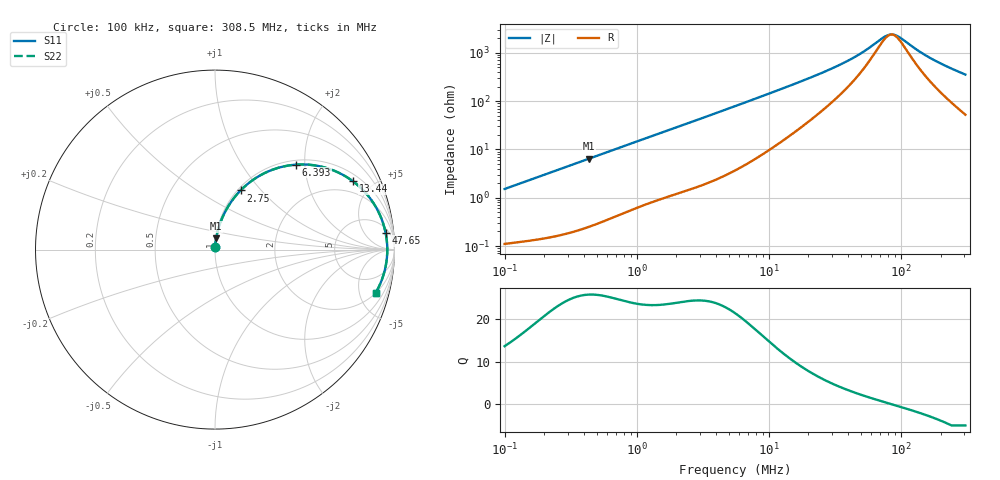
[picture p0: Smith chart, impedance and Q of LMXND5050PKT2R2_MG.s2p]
! LMXND5050PKT2R2_MG  S-PARAMETER MODEL  ( General Type )
! Model Generated by TAIYO YUDEN Corporation (https://www.yuden.co.jp/en/)
! Version 1.0
! TAIYO YUDEN Control No. 191023NI43SB-FBB
! Copyright(c) 2019 TAIYO YUDEN CO.,LTD. All Rights Reserved.
! Product Description (link to TY-COMPAS)
! https://ds.yuden.co.jp/TYCOMPAS/or/detail?pn=LMXND5050PKT2R2NMG&u=M
! Products Name : Inductors
! Characteristics :
!  Inductance : 2.2 uH , SRF(min) : 56 MHz , DC Resistance(max) : 0.078 Ohm
!  Rated Current : Saturation :2800 mA , Temp Rise : 2000 mA (40 degC)
!  Case Size : 4.9 x 4.9 / 0.193 x 0.193 [mm/inch] , Thickness : 1.4 / 0.055 [mm/inch]
!  (Conditions: Temperature = 25 degC , DC Bias Current/Voltage = 0A / 0V)
! External Node Assignments :
!  1  o---GGG---o  2
! GND o---------o GND
! Frequency Range : 0.1MHz  -  308.54851MHz  [ 402 STEP ]
# MHz S RI R 50
! Freq[MHz].  S11 Real  S11 Imag  S21 Real  S21 Imag  S12 Real  S12 Imag  S22 Real  S22 Imag
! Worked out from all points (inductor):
!   401 points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, 100 kHz to 308.5 MHz, reference 50 ohm
!   read as one part in series: L = 2.39 uH near 104.1 kHz
!   highest Q = 25.8 at 433.3 kHz (marker M1), where L = 2.36 uH
!   self-resonance near 85.23 MHz
!   S11 on the Smith chart (normalised r, x): 100 kHz: 1.00, +0.03; 2.75 MHz: 1.03, +0.78; 6.393 MHz: 1.09, +1.81; 13.44 MHz: 1.33, +3.85; 47.65 MHz: 8, +17; 308.5 MHz: 2.05, -7.00
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0.1  0.00133 0.0151  0.9987 -0.0151  0.9987 -0.0151  0.00133 0.0151
0.384115  0.00543 0.0565  0.9946 -0.0565  0.9946 -0.0565  0.00543 0.0565
0.433313  0.00654 0.0635  0.9935 -0.0635  0.9935 -0.0635  0.00654 0.0635
0.824038  0.019 0.1176  0.981 -0.1176  0.981 -0.1176  0.019 0.1176
1.475446  0.0509 0.1995  0.9491 -0.1995  0.9491 -0.1995  0.0509 0.1995
2.750084  0.1421 0.3293  0.8579 -0.3293  0.8579 -0.3293  0.1421 0.3293
3.947894  0.2467 0.4106  0.7533 -0.4106  0.7533 -0.4106  0.2467 0.4106
5.667415  0.3956 0.4661  0.6044 -0.4661  0.6044 -0.4661  0.3956 0.4661
6.393297  0.4521 0.4734  0.5479 -0.4734  0.5479 -0.4734  0.4521 0.4734
8.995414  0.613 0.457  0.387 -0.457  0.387 -0.457  0.613 0.457
13.44272  0.7694 0.3801  0.2306 -0.3801  0.2306 -0.3801  0.7694 0.3801
21.33651  0.8798 0.2638  0.1202 -0.2638  0.1202 -0.2638  0.8798 0.2638
33.19221  0.9312 0.1625  0.0688 -0.1625  0.0688 -0.1625  0.9312 0.1625
47.64921  0.9505 0.0937  0.0495 -0.0937  0.0495 -0.0937  0.9505 0.0937
72.65161  0.9593 0.0247  0.0407 -0.0247  0.0407 -0.0247  0.9593 0.0247
81.95682  0.9599 0.00602  0.0401 -0.00602  0.0401 -0.00602  0.9599 0.00602
87.04724  0.9599 -0.00326  0.0401 0.00326  0.0401 0.00326  0.9599 -0.00326
94.32966  0.9597 -0.0156  0.0403 0.0156  0.0403 0.0156  0.9597 -0.0156
135.4153  0.9543 -0.0734  0.0457 0.0734  0.0457 0.0734  0.9543 -0.0734
165.5392  0.9476 -0.1085  0.0524 0.1085  0.0524 0.1085  0.9476 -0.1085
228.2831  0.9283 -0.1716  0.0717 0.1716  0.0717 0.1716  0.9283 -0.1716
308.5485  0.8956 -0.2401  0.1044 0.2401  0.1044 0.2401  0.8956 -0.2401
